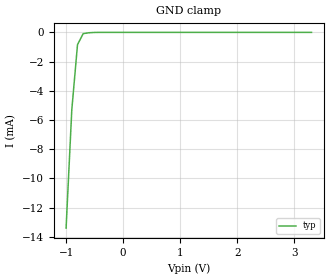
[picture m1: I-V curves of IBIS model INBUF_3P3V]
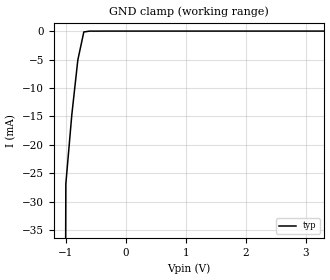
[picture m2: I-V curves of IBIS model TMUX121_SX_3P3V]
|Texas Instruments Incorporated
| IBIS Model of : TMUX121
| 3.3V 2x1:2 Analog Switch Array
| This file contains package information for the following:
|  UQFN 10-pin (NKG) package as [Component] TMUX121
| This device can be powered at the following Vccs:
| Single Rail Supply Configurations:
|  3.3 volt VCC
| Digital Voltage Range : 3.0-3.6
[IBIS Ver] 4.1
[File name] TMUX121.ibs
[File Rev] 1.0
[Date] 11/15/2023
[Source]
| Texas Instruments Incorporated.
| 12500 TI Blvd
| Dallas, TX -75243
[Notes] Revision History:
| Rev 1.0: 11/15/2023
| - Initial version of the model
| - Model generated from bench measurements of nominal silicon
| - C_comp although listed in numerical order of value are
| obtained from varying PVT conditions. For PVT conditions for
| each specific value refer the buffer description under
| respective [Model]. IBIS model user is responsible for using
| appropriate C_comp to simulate for Signal Integrity.
| - Warnings regarding combined Non-monotonicity of various models have been
| reviewed and considered minor and can be ignored.
|**** Modify the following if you use [Model Selector]***********
| - Model names with a trailing voltage extension contain the model for
| operation at that voltage range.
[Disclaimer]
| This model is designed as an aid for customers of Texas Instruments.
| TI and its licensors and suppliers make no warranties, either expressed
| or implied, with respect to this model, including the warranties of
| merchantability or fitness for a particular purpose. The model is
| provided solely on an "as is" basis. The entire risk as to its quality
| and performance is with the customer.
| This model is subject to change without notice. Texas Instruments
| Incorporated is not responsible for updating this model.
[Copyright]
(C) Copyright 2023 Texas Instruments Incorporated. All rights reserved.
| Component TMUX121 10-pin UQFN (per package)
[Component] TMUX121
[Manufacturer]  Texas Instruments Incorporated
[Package] |UQFN (NKG) 10-pin
| variable typ min max
R_pkg 0.05 0.04 0.06
L_pkg 1.0nH 0.8nH 1.2nH
C_pkg 0.2pF 0.16pF 0.24pF
| pin number (pin name) mapping to model name
[Pin] signal_name   model_name   R_pin L_pin C_pin
1   D1 	TMUX121_DX   NA   NA   NA
2   D2   TMUX121_DX   NA   NA   NA
3   S1A  	TMUX121_SX   NA   NA   NA
4   S2A   TMUX121_SX   NA   NA   NA
5   S1B 	TMUX121_SX   NA   NA   NA
6   S2B  	TMUX121_SX   NA   NA   NA
7   SEL	INPUT_BUF		NA   NA   NA
8   ENZ	INPUT_BUF		NA   NA   NA
9   VDD	POWER			NA   NA   NA
10   GND   GND		NA   NA   NA
[Series Switch Groups]
| Function Group States
On  1 /   | ENZ LOW, SEL LOW -> D1 to S1A, D2 to S2A
On  2 /   | ENZ LOW, SEL HIGH -> D1 to S1B, D2 to S2B
Off  /   | ENZ HIGH
[Series Pin Mapping]   pin_2   model_name   function_table_group
| PW Package
1   3   TMUX121_SX_3P3V_S   1
|3   1   TMUX121_DX_3P3V_S   1
|2   4   TMUX121_SX_3P3V_S   1
|4   2   TMUX121_DX_3P3V_S   1
|1   5   TMUX121_SX_3P3V_S   2
|5   1   TMUX121_DX_3P3V_S   2
|2   6   TMUX121_SX_3P3V_S   2
|6   2   TMUX121_DX_3P3V_S   2
| Model Selectors
|*** power supply options or driver programmability *********
[Model Selector] INPUT_BUF
INBUF_3P3V   buffer at 3P3V operation.
[Model Selector] TMUX121_SX
TMUX121_SX_3P3V  switch termination at +3.3V operation.
[Model Selector] TMUX121_DX
TMUX121_DX_3P3V  termination switch at +3.3V operation.
| Model2
[Model]   TMUX121_SX_3P3V_S
Model_type  Series_switch
| variable   typ   min   max
C_comp   1.7pF   NA   NA
[Temperature Range]   25   NA   NA
| Ambient temperature   25   NA   NA
[Voltage range]   3.3   NA   NA
[On]
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[Off]
|   typ   min   max
[R Series]   10G   NA   NA
[Model]   TMUX121_DX_3P3V_S
Model_type  Series_switch
| variable   typ   min   max
C_comp   1.7pF		NA   NA
[Temperature Range]   25   NA   NA
| Ambient temperature   25   NA   NA
[Voltage range]   3.3   NA   NA
[On]
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[Off]
|   typ   min   max
[R Series]   10G   NA   NA
| Models and submodels in the file (5): INBUF_3P3V (Input), TMUX121_SX_3P3V_S (Series_switch), TMUX121_SX_3P3V (Terminator), TMUX121_DX_3P3V_S (Series_switch), TMUX121_DX_3P3V (Terminator)
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| Model1
[Model]   INBUF_3P3V
Model_type   Input
Vinl = 0.4
Vinh = 1.4
|   typ   min   max
C_comp   3pF   NA		NA
[Voltage Range]   3.3   NA		NA
[Temperature Range]   27   NA		NA
[Power Clamp Reference]   3.3   NA		NA
[GND Clamp Reference]   0   NA		NA
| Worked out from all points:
|   GND clamp passes 1 mA (typ) near -0.80 V on its own axis
[GND Clamp]
|   Voltage   I(typ)   I(min)   I(max)
-1V       -13.4mA    NA         NA
-900mV    -5.3mA     NA         NA
-800mV    -840uA     NA         NA
-700mV    -85uA      NA         NA
-400mV    -500nA     NA         NA
3.3V      0A         NA         NA
[POWER Clamp]
|   Voltage   I(typ)   I(min)   I(max)
-3.3V     0A         NA         NA
-3.1V     0A         NA         NA
-2.9V     0A         NA         NA
3.3V      0A         NA         NA
[Model]   TMUX121_SX_3P3V
Model_type   Terminator
|   typ   min   max
C_comp   0pF   NA   NA
[Voltage Range]   3.3   NA   NA
[Temperature Range]   27   NA   NA
[Power Clamp Reference]   3.3   NA   NA
[GND Clamp Reference]   0   NA   NA
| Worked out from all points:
|   GND clamp passes 1 mA (typ) near -0.72 V on its own axis
[GND Clamp]
|   Voltage   I(typ)   I(min)   I(max)
-1.2V     -52.7mA    NA         NA
-1.1V     -401mA     NA         NA
-1V       -26.9mA    NA         NA
-900mV    -14.7mA    NA         NA
-800mV    -5.1mA     NA         NA
-700mV    -153uA     NA         NA
-600mV    -1.6uA     NA         NA
3.3V      0A         NA         NA
[POWER Clamp]
|   Voltage   I(typ)   I(min)   I(max)
-3.3V     0A         NA         NA
-3.1V     0A         NA         NA
-2.9V     0A         NA         NA
3.3V      0A         NA         NA
